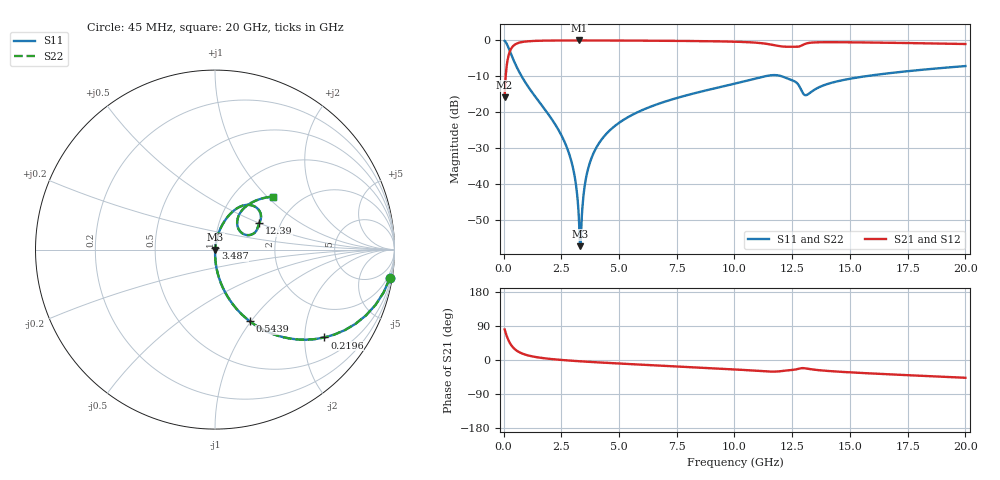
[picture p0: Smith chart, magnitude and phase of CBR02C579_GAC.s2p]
! S-parameter model data by Modelithics Inc.  support@modelithics.com 813-866-6335  Tampa FL USA
! S-Parameter data specifications:
! Substrate: 20-mil Rogers 4350B, substrate thickness, H=0.508mm, Dielectric constant, Er=3.75
! PCB Mounting Pad Footprint: Pad width, PadW=0.32mm , Pad length, PadL=0.37mm , Pad gap, PadG (edge-to-edge)=0.19mm , Reference planes=0.93mm apart
#  GHz  S  MA  R 50
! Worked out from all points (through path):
!   801 points, 45 MHz to 20 GHz, reference 50 ohm
!   highest |S21| = -0.01 dB at 3.263 GHz (marker M1); lowest = -15.9 dB at 45 MHz (marker M2)
!   group delay of S21, straight-line fit = 8.38 ps
!   lowest |S11| = -57.3 dB at 3.313 GHz (marker M3), VSWR 1.00, Z = 50.1 - j0.0579 ohm
!   |S11| at or under -10 dB: 783.5 MHz to 11.31 GHz (10.52 GHz wide, 174 % of centre); 12.05 GHz to 15.65 GHz (3.592 GHz wide, 25.9 % of centre)
!   |S22| runs from -57.3 to -0.1 dB; largest |S21 - S12| = 0
!   S11 on the Smith chart (normalised r, x): 45 MHz: 1, -12; 219.6 MHz: 0.99, -2.50; 543.9 MHz: 0.99, -0.99; 3.487 GHz: 1.00, +0.02; 12.39 GHz: 1.56, +0.50; 20 GHz: 1.49, +1.09
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0.045  0.987 -9.3  0.1606 80.7  0.1606 80.7  0.987 -9.3
0.219606  0.7816 -38.8  0.6232 51.2  0.6232 51.2  0.7816 -38.8
0.543875  0.4434 -64.1  0.8955 25.8  0.8955 25.8  0.4434 -64.1
1.142525  0.2088 -78.9  0.977 10.9  0.977 10.9  0.2088 -78.9
2.689037  0.03567 -88.8  0.9981 -0.8  0.9981 -0.8  0.03567 -88.8
3.063194  0.0137 -87.2  0.9986 -2.4  0.9986 -2.4  0.0137 -87.2
3.262744  0.003303 -70.6  0.9987 -3.2  0.9987 -3.2  0.003303 -70.6
3.312631  0.00137 -24.9  0.9987 -3.4  0.9987 -3.4  0.00137 -24.9
3.387462  0.003493 64.8  0.9987 -3.7  0.9987 -3.7  0.003493 64.8
3.487237  0.008235 76.9  0.9986 -4.1  0.9986 -4.1  0.008235 76.9
3.611956  0.01412 80.1  0.9985 -4.6  0.9985 -4.6  0.01412 80.1
3.786563  0.02211 81.4  0.9984 -5.2  0.9984 -5.2  0.02211 81.4
4.335325  0.04549 81.1  0.9975 -7.1  0.9975 -7.1  0.04549 81.1
5.283188  0.08169 78.8  0.995 -10.2  0.995 -10.2  0.08169 78.8
6.704981  0.1311 74.7  0.9894 -14.5  0.9894 -14.5  0.1311 74.7
10.0225  0.2508 63.1  0.9593 -24.9  0.9593 -24.9  0.2508 63.1
11.6189  0.3283 45.9  0.8714 -30.7  0.8714 -30.7  0.3283 45.9
12.39216  0.2865 30.7  0.8165 -26.8  0.8165 -26.8  0.2865 30.7
13.04069  0.1742 33.6  0.8904 -21.8  0.8904 -21.8  0.1742 33.6
13.36496  0.1962 51.0  0.9335 -24.8  0.9335 -24.8  0.1962 51.0
16.68248  0.3492 50.7  0.9274 -37.8  0.9274 -37.8  0.3492 50.7
20  0.4398 42.2  0.8911 -46.9  0.8911 -46.9  0.4398 42.2
